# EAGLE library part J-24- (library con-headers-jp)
HEADER JACK PINS
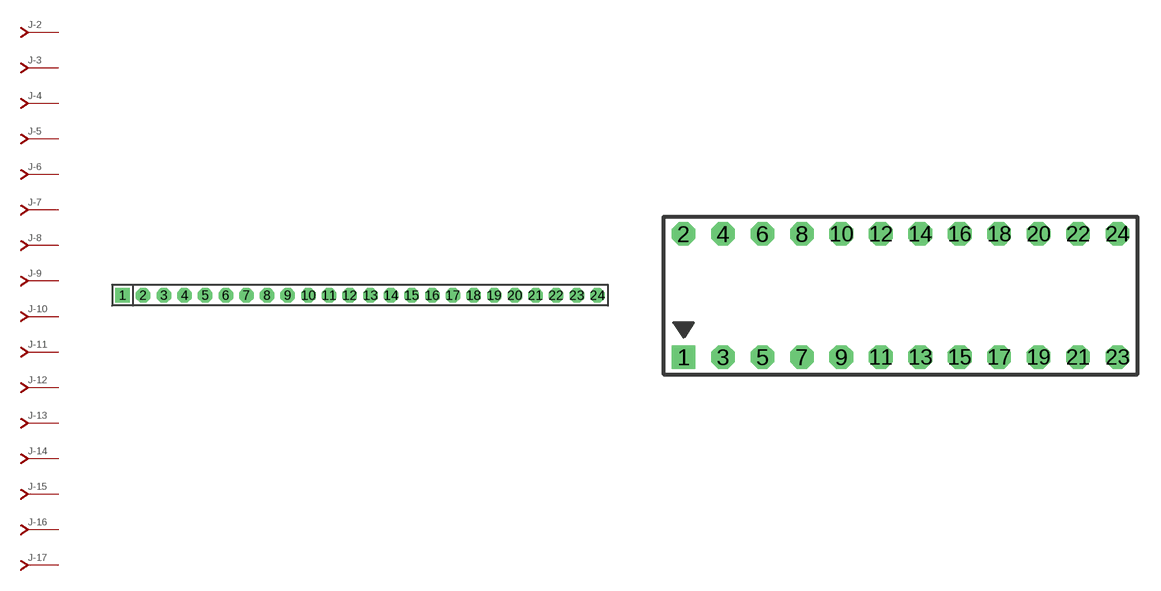
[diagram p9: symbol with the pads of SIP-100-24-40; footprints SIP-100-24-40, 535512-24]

Designator prefix J; gates -2=J-N -3=J-N -4=J-N -5=J-N -6=J-N -7=J-N -8=J-N -9=J-N -10=J-N -11=J-N -12=J-N -13=J-N -14=J-N -15=J-N -16=J-N -17=J-N -18=J-N -19=J-N -20=J-N -21=J-N -22=J-N -23=J-N -24=J-N -1=J-NV

## J-24-SIP-100-40  [SIP-100-24-40]
1  -1:J  pas
2  -2:J  pas
3  -3:J  pas
4  -4:J  pas
5  -5:J  pas
6  -6:J  pas
7  -7:J  pas
8  -8:J  pas
9  -9:J  pas
10  -10:J  pas
11  -11:J  pas
12  -12:J  pas
13  -13:J  pas
14  -14:J  pas
15  -15:J  pas
16  -16:J  pas
17  -17:J  pas
18  -18:J  pas
19  -19:J  pas
20  -20:J  pas
21  -21:J  pas
22  -22:J  pas
23  -23:J  pas
24  -24:J  pas

## J-24-535512  [535512-24]
Pads as for SIP-100-24-40

## J-24-79107  [79107-24]
Pads as for SIP-100-24-40

## J-24-79109  [79109-24]
Pads as for SIP-100-24-40

## J-24-87264  [87264-24]
Pads as for SIP-100-24-40

## J-24-87368  [87368-24]
Pads as for SIP-100-24-40

## J-24-100-2X12  [DIL-100-2X12]
Pads as for SIP-100-24-40

## J-24-100-2X12_M  [DIL-100-2X12_M]
Pads as for SIP-100-24-40

## J-24-2MM-2X12  [DIL-2MM-2X12]
Pads as for SIP-100-24-40

## J-24-2MM-2X12_M  [DIL-2MM-2X12_M]
Pads as for SIP-100-24-40

## J-24-SIP-100-32  [SIP-100-24-32]
Pads as for SIP-100-24-40

## J-24-SIP-100-40Y  [SIP-100-24-40Y]
Pads as for SIP-100-24-40

## J-24-SIP-100-32Y  [SIP-100-24-32Y]
Pads as for SIP-100-24-40

## J-24-71991  [71991-24]
Pads as for SIP-100-24-40

## J-24-KK-4455-B24  [KK-4455-B24]
Pads as for SIP-100-24-40

## J-24-KK-4455-A24  [KK-4455-A24]
Pads as for SIP-100-24-40

## J-24-KK-4455-C24  [KK-4455-C24]
Pads as for SIP-100-24-40

## Footprint SIP-100-24-40 (pad centres in mm)
SIP Header - 0.1", 40 mil drill
drill 1.016 pad 1.778 square: 1 -29.21,0
drill 1.016 pad 1.778 octagon: 2 -26.67,0; 3 -24.13,0; 4 -21.59,0; 5 -19.05,0; 6 -16.51,0; 7 -13.97,0; 8 -11.43,0; 9 -8.89,0; 10 -6.35,0; 11 -3.81,0; 12 -1.27,0; 13 1.27,0; 14 3.81,0; 15 6.35,0; 16 8.89,0; 17 11.43,0; 18 13.97,0; 19 16.51,0; 20 19.05,0; 21 21.59,0; 22 24.13,0; 23 26.67,0; 24 29.21,0

## Footprint 535512-24 (pad centres in mm)
AMPMODU - 535512 Series
drill 1.016 square: 1 -13.97,0
drill 1.016 octagon: 2 -13.97,7.938; 3 -11.43,0; 4 -11.43,7.938; 5 -8.89,0; 6 -8.89,7.938; 7 -6.35,0; 8 -6.35,7.938; 9 -3.81,0; 10 -3.81,7.938; 11 -1.27,0; 12 -1.27,7.938; 13 1.27,0; 14 1.27,7.938; 15 3.81,0; 16 3.81,7.938; 17 6.35,0; 18 6.35,7.938; 19 8.89,0; 20 8.89,7.938; 21 11.43,0; 22 11.43,7.938; 23 13.97,0; 24 13.97,7.938

## Footprint 79107-24 (pad centres in mm)
Molex Board-To-Board Receptacal 2.00mm (.079") Pitch Milli-Grid Header, Vertical, Through-Hole Mates with: 87759, 87762, 87758, 87760
drill 0.711 square: 1 -11,-1
drill 0.711: 2 -11,1; 3 -9,-1; 4 -9,1; 5 -7,-1; 6 -7,1; 7 -5,-1; 8 -5,1; 9 -3,-1; 10 -3,1; 11 -1,-1; 12 -1,1; 13 1,-1; 14 1,1; 15 3,-1; 16 3,1; 17 5,-1; 18 5,1; 19 7,-1; 20 7,1; 21 9,-1; 22 9,1; 23 11,-1; 24 11,1

## Footprint 79109-24 (pad centres in mm)
Molex Board-to-Board Receptacal 2.00mm (.079") Pitch Milli-Grid Header, Vertical, Top/Bottom Entry Mates with: 87758, 87759, 87760, 87831, 87832, 87833
smd 1.12 x 1.83: 1 -11,-2.65; 2 -11,2.65; 3 -9,-2.65; 4 -9,2.65; 5 -7,-2.65; 6 -7,2.65; 7 -5,-2.65; 8 -5,2.65; 9 -3,-2.65; 10 -3,2.65; 11 -1,-2.65; 12 -1,2.65; 13 1,-2.65; 14 1,2.65; 15 3,-2.65; 16 3,2.65; 17 5,-2.65; 18 5,2.65; 19 7,-2.65; 20 7,2.65; 21 9,-2.65; 22 9,2.65; 23 11,-2.65; 24 11,2.65
hole 0.914 at -10,0
hole 0.914 at -11,1
hole 0.914 at -11,-1
hole 0.914 at -9,-1
hole 0.914 at -9,1
hole 0.914 at -7,-1
hole 0.914 at -7,1
hole 0.914 at 10,0
hole 0.914 at -5,1
hole 0.914 at -5,-1
hole 0.914 at -3,1
hole 0.914 at -3,-1
hole 0.914 at -1,1
hole 0.914 at -1,-1
hole 0.914 at 1,1
hole 0.914 at 1,-1
hole 0.914 at 3,-1
hole 0.914 at 3,1
hole 0.914 at 5,1
hole 0.914 at 5,-1
hole 0.914 at 7,1
hole 0.914 at 7,-1
hole 0.914 at 9,1
hole 0.914 at 9,-1
hole 0.914 at 11,-1
hole 0.914 at 11,1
